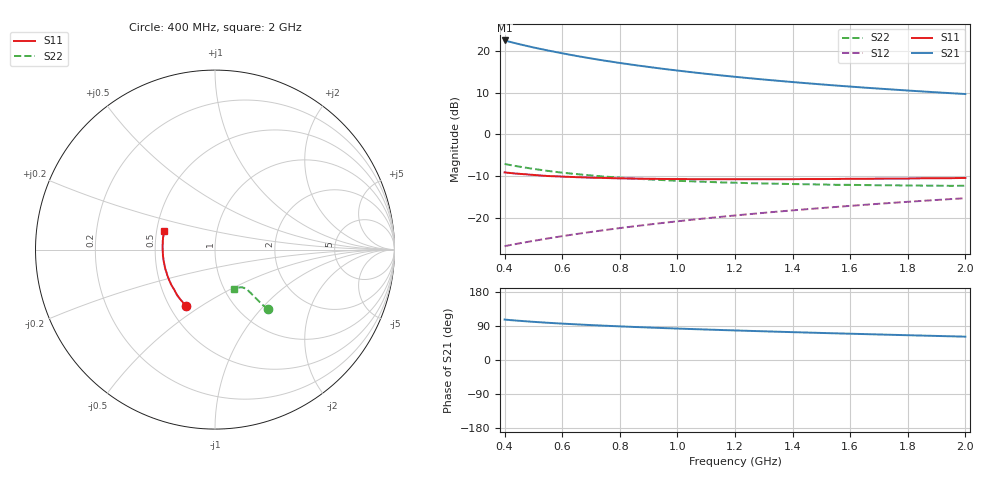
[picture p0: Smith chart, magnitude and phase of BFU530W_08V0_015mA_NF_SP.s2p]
! Filename:  P:\Prog\Test\Noise\ATS_data\Testdata_Net\06 Compressed Noise after Statistics\BFU530W_APM2013_09_A05_08p0V_015mA_NF_CM01_D.sf
! Date/Time: Tue 26/Mar/2013 18:06:03
! BFU530W_APM2013_09_A05_08p0V_1to25mA_NF_CM01_Bias7_R.sf
! Noise Parameter Data File
! BFU530W_APM2013_09_A05_08p0V_1to25mA_NF_CM01
! Date/time: Thu Mar 21 21:44:48 2013
! VAR V_out= 8.000000
! VAR I_out= 14.990000
! VAR V_in= 0.812800
! VAR I_in= 0.151400
! Device data file deembeded for feedlines and parallel
! Original file: \06 Compressed Noise after Statistics\BFU530W_APM2013_09_A05_08p0V_015mA_NF_CM01_R.sf
! Feed-files: PR019V01_070313_Feed1.s2p, PR019V01_070313_Feed2.s2p
! Parallel-file: PR019V01_070313_Par.s2p
# MHz S MA R 50
!  Freq-MHz  S11-mag  S11-arg  S21-mag  S21-arg  S12-mag  S12-arg  S22-mag  S22-arg
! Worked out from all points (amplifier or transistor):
!   37 points, 400 MHz to 2 GHz, reference 50 ohm
!   highest |S21| = 22.4 dB at 400 MHz (marker M1)
!   |S21| within 3 dB of that: start of sweep to 595.2 MHz
!   unconditionally stable (mu >= 1): 1.229 GHz to end of sweep
!   at 500 MHz: K = 0.82, MSG = 23.1 dB, |S12| = -25.4 dB
!   at 1.1 GHz: K = 0.99, MSG = 17.2 dB, |S12| = -20.0 dB
!   at 2 GHz: K = 1.01, MAG = 11.7 dB, |S12| = -15.2 dB
!   lowest NFmin = 0.89 dB at 400 MHz
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400  0.352 -117.7  13.24 106.7  0.04632 62.9  0.4439 -48.4
420  0.3462 -120.6  12.71 105.3  0.04781 63.0  0.4308 -48.7
433  0.3421 -122.3  12.38 104.5  0.04871 63.2  0.4225 -48.9
460  0.3366 -125.6  11.75 102.9  0.0507 63.5  0.408 -49.2
500  0.3284 -130.5  10.93 100.7  0.05355 63.9  0.3875 -49.5
550  0.3186 -135.4  10.05 98.2  0.05727 64.6  0.3671 -49.8
600  0.3139 -140.3  9.301 96.0  0.061 65.0  0.3494 -50.0
650  0.3087 -144.5  8.646 94.0  0.06472 65.5  0.3358 -50.2
700  0.3046 -148.4  8.075 92.1  0.06846 66.0  0.3237 -50.4
750  0.3018 -151.8  7.574 90.4  0.0723 66.4  0.3131 -50.5
800  0.2984 -155.2  7.133 88.8  0.07614 66.7  0.3052 -50.8
850  0.2972 -158.4  6.741 87.2  0.07998 67.0  0.2968 -50.9
950  0.2939 -163.7  6.074 84.3  0.08784 67.4  0.2849 -51.4
1050  0.2925 -168.6  5.529 81.7  0.09572 67.7  0.2755 -52.0
1150  0.2921 -173.2  5.072 79.2  0.1036 67.8  0.2675 -52.7
1200  0.2912 -175.2  4.877 78.0  0.1077 67.8  0.2653 -53.3
1250  0.2914 -177.2  4.69 76.8  0.1117 67.8  0.2619 -53.7
1350  0.2915 179.3  4.367 74.6  0.1199 67.7  0.2579 -54.7
1500  0.293 174.1  3.955 71.4  0.1321 67.4  0.2525 -56.7
1650  0.295 169.3  3.619 68.4  0.1444 67.0  0.2484 -58.6
1750  0.2971 166.6  3.431 66.4  0.1527 66.6  0.2469 -60.0
2000  0.3024 159.9  3.035 61.6  0.1733 65.4  0.2437 -64.1
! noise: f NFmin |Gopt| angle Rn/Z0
400  0.891  0.1541  179.4  0.0853
460  0.9022  0.1635  -178  0.0819
600  0.9067  0.1704  -176.1  0.0839
800  0.9604  0.1844  -175.4  0.0793
1000  0.9858  0.2037  -172.4  0.0759
1200  1.029  0.2012  -168.2  0.0819
1400  1.047  0.2337  -164.3  0.0747
1600  1.067  0.2531  -162.9  0.0718
1800  1.079  0.2676  -158.1  0.074
2000  1.116  0.2772  -154.2  0.0818
